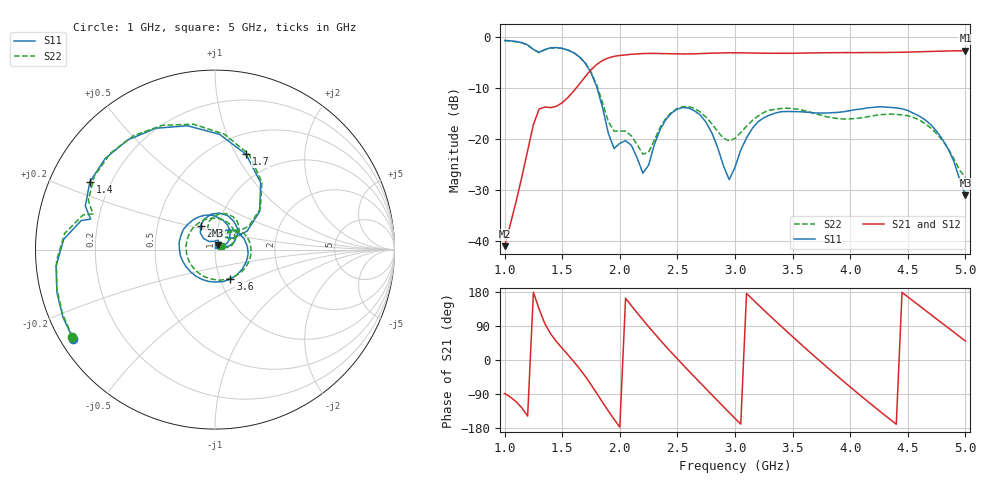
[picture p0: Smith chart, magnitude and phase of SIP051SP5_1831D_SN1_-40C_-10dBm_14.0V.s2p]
# GHz  S  dB  R  50
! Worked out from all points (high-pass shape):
!   81 points, 1 GHz to 5 GHz, reference 50 ohm
!   highest |S21| = -2.61 dB at 5 GHz (marker M1); lowest = -41.0 dB at 1 GHz (marker M2)
!   |S21| within 3 dB of the highest: 1.785 GHz to end of sweep
!   lowest |S11| = -31.0 dB at 5 GHz (marker M3), VSWR 1.06, Z = 51.6 + j2.39 ohm
!   |S11| at or under -10 dB: 1.804 GHz to end of sweep
!   |S22| runs from -27.4 to -0.6 dB; largest |S21 - S12| = 0.0021
!   S11 on the Smith chart (normalised r, x): 1 GHz: 0.04, -0.29; 1.4 GHz: 0.12, +0.25; 1.7 GHz: 0.71, +1.10; 2.4 GHz: 0.82, +0.23; 3.6 GHz: 1.12, -0.38; 5 GHz: 1.03, +0.05
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1  -0.59 -147.7  -41.00 -88.5  -40.97 -88.9  -0.62 -148.6
1.25  -2.35 167.8  -17.10 178.6  -17.15 178.8  -2.38 165.3
1.4  -2.02 151.6  -13.78 68.9  -13.80 68.9  -2.08 148.7
1.55  -2.47 116.0  -11.78 13.6  -11.77 13.7  -2.47 113.0
1.7  -5.06 71.9  -7.69 -43.0  -7.69 -43.1  -4.99 70.3
1.85  -13.75 29.9  -4.52 -111.4  -4.51 -111.3  -12.80 34.7
2  -20.80 76.0  -3.53 -177.2  -3.53 -177.2  -18.37 63.9
2.2  -26.66 90.2  -3.16 106.1  -3.17 106.1  -22.92 75.1
2.35  -18.10 131.0  -3.16 52.8  -3.15 52.9  -17.66 108.0
2.4  -16.13 120.7  -3.18 35.8  -3.18 35.8  -15.88 102.0
2.55  -13.76 83.0  -3.24 -13.3  -3.22 -13.3  -13.58 72.3
2.75  -16.72 32.3  -3.13 -76.5  -3.13 -76.5  -15.69 35.8
2.95  -27.94 44.2  -3.01 -138.7  -3.01 -138.8  -20.32 41.5
3  -25.49 71.7  -3.02 -154.1  -3.01 -154.0  -19.84 49.3
3.15  -17.88 58.7  -3.06 160.9  -3.06 160.9  -16.30 45.5
3.35  -14.85 6.4  -3.11 103.3  -3.11 103.3  -14.10 11.8
3.6  -14.65 -62.6  -3.06 34.2  -3.06 34.2  -14.36 -42.6
3.7  -14.85 -88.8  -3.03 7.3  -3.03 7.3  -15.00 -68.2
4.05  -14.16 -169.9  -2.98 -83.8  -2.95 -83.8  -15.93 -171.8
4.35  -13.74 126.4  -2.93 -157.6  -2.95 -157.6  -15.07 105.7
4.7  -17.13 54.7  -2.74 119.9  -2.74 119.9  -17.79 30.9
5  -30.97 55.0  -2.61 50.2  -2.62 50.2  -27.45 31.9
